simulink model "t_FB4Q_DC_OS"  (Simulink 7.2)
settings: Solver=ode3  SolverMode=SingleTasking  StartTime=0.0  StopTime=0.02  FixedStep=10e-6  MaxStep=5e-6  RelTol=1e-6  AbsTol=1e-6

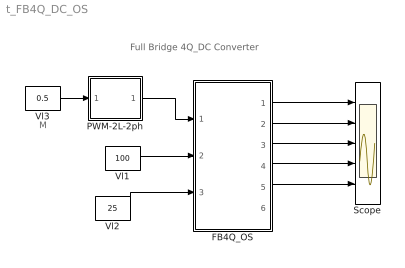
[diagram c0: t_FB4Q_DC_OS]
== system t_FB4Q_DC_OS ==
  note: Full Bridge 4Q_DC Converter
  note: M
  FB4Q_OS : Subsystem  mask{L=5e-3, IL0=30, C=2e-4, VC0=50, R=10}
      mask prompts: L "Inductance L"; IL0 "Initial Current"; C "Cap"; VC0 "Initial Cap Voltage"; R "Load Resistance"
      mask help: Full Bridge 4Q Converter Input Vector u: u[0]= T1.gate u[1]= T2.gate u[2]= T3.gate u[3]= T4.gate u[4]= E.V u[5]= IDC.i Output Vector y: y[0]= T1.I y[1]= D1.I y[2]= T3.I y[3]= D3.I y[4]= Vo.V y[5]= L1.I y[6]= C1.V y[7]= E.I Parameter Vector p: p[0]= L1.L p[1]= L1.iL0 p[2]= C1.C p[3]= C1.vC0 p[4]= R1.r You can pause the simulation during running, change the Parameters you want and continue the Simulation
  PWM-2L-2ph : Subsystem  mask(PWM-2L-2PH){FT=500, PHT=0, DT=1e-6}
      mask prompts: FT "Triangular Frequency"; PHT "Trian. Phase Angle (Degree)"; DT "Dead Time"
  Scope : Scope  NumInputPorts=5
  Vl1 : Constant  Value=100
  Vl2 : Constant  Value=25
  Vl3 : Constant  Value=0.5
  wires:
  FB4Q_OS/1("iT1, iD1") -> Scope/1
  PWM-2L-2ph/1(O1) -> FB4Q_OS/1(sw)
  Vl1/1 -> FB4Q_OS/2(E)
  Vl2/1 -> FB4Q_OS/3(ID)
  FB4Q_OS/4(iL) -> Scope/4
  FB4Q_OS/3(vO) -> Scope/3
  Vl3/1 -> PWM-2L-2ph/1(I1)
  FB4Q_OS/2("iT3, iD3") -> Scope/2
  FB4Q_OS/5(vC) -> Scope/5

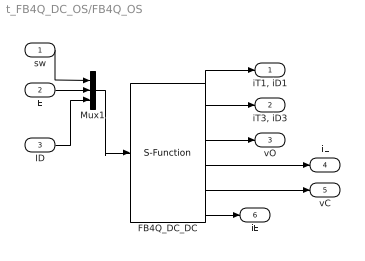
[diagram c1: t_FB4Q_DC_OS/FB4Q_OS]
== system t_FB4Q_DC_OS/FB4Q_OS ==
  sw : Inport  OutDataType=sfix(16)  OutScaling=2^0
  E : Inport  Port=2  OutDataType=sfix(16)  OutScaling=2^0
  ID : Inport  Port=3  OutDataType=sfix(16)  OutScaling=2^0
  FB4Q_DC_DC : S-Function  FunctionName=s_FB4Q_DC_OS  Parameters="[L  IL0  C  VC0   R]"  EnableBusSupport=off
  Mux1 : Mux  Inputs=3
  "iT1, iD1" : Outport  OutDataType=sfix(16)  OutScaling=2^0
  "iT3, iD3" : Outport  Port=2  OutDataType=sfix(16)  OutScaling=2^0
  vO : Outport  Port=3  OutDataType=sfix(16)  OutScaling=2^0
  iL : Outport  Port=4  OutDataType=sfix(16)  OutScaling=2^0
  vC : Outport  Port=5  OutDataType=sfix(16)  OutScaling=2^0
  iE : Outport  Port=6  OutDataType=sfix(16)  OutScaling=2^0
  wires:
  Mux1/1 -> FB4Q_DC_DC/1
  sw/1 -> Mux1/1
  E/1 -> Mux1/2
  FB4Q_DC_DC/1 -> "iT1, iD1"/1
  FB4Q_DC_DC/2 -> "iT3, iD3"/1
  ID/1 -> Mux1/3
  FB4Q_DC_DC/4 -> iL/1
  FB4Q_DC_DC/3 -> vO/1
  FB4Q_DC_DC/5 -> vC/1
  FB4Q_DC_DC/6 -> iE/1

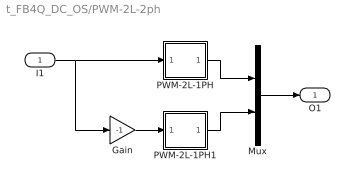
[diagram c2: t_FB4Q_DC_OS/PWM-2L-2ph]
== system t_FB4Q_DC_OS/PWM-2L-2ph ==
  I1 : Inport  OutDataType=sfix(16)  OutScaling=2^0
  Gain : Gain  Gain=-1  ParameterDataType=sfix(16)  ParameterScaling=2^0  OutDataType=sfix(16)  OutScaling=2^0
  Mux : Mux  Inputs=2
  PWM-2L-1PH : Subsystem  mask(PWM-2L-1PH){FT=FT, PHT=PHT, DT=DT}
      mask prompts: FT "Triangular Frequency"; PHT "Trian. Phase Angle (Degree)"; DT "Dead Time"
      mask help: Pulse Width Modulation for 1 Phase Converter
  PWM-2L-1PH1 : Subsystem  mask(PWM-2L-1PH){FT=FT, PHT=PHT, DT=DT}
      mask prompts: FT "Triangular Frequency"; PHT "Trian. Phase Angle (Degree)"; DT "Dead Time"
      mask help: Pulse Width Modulation for 1 Phase Converter
  O1 : Outport
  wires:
  Gain/1 -> PWM-2L-1PH1/1(In1)
  I1/1 -> Gain/1, PWM-2L-1PH/1(In1)
  PWM-2L-1PH/1(Out1) -> Mux/1
  PWM-2L-1PH1/1(Out1) -> Mux/2
  Mux/1 -> O1/1

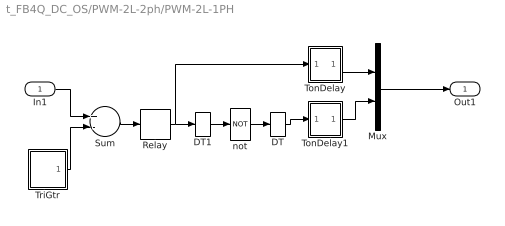
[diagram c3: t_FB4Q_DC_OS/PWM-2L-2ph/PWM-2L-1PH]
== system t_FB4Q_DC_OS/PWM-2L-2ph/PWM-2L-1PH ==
  In1 : Inport  OutDataType=sfix(16)  OutScaling=2^0
  DT : DataTypeConversion
  DT1 : DataTypeConversion
  Mux : Mux  Inputs=2
  Relay : Relay  OutDataType=sfix(16)  OutScaling=2^0
  Sum : Sum  Inputs=+-  OutDataType=sfix(16)  OutScaling=2^0
  TonDelay : Subsystem  mask(TonDelay){DT=DT}
      mask prompts: DT "Dead Time"
      mask help: Turn on dead time to protect against short circuit of the converter leg
  TonDelay1 : Subsystem  mask(TonDelay){DT=DT}
      mask prompts: DT "Dead Time"
      mask help: Turn on dead time to protect against short circuit of the converter leg
  TriGtr : Subsystem  mask(TriGtr){T=1/FT, Td=PHT/FT/360}
      mask prompts: T "Period Time"; Td "Time Delay"
      mask help: Triangular Wave Generator with variable time delay
  not : Logic  Operator=NOT  Inputs=1
  Out1 : Outport  InitialOutput=0
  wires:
  DT1/1 -> not/1
  DT/1 -> TonDelay1/1(s1)
  In1/1 -> Sum/1
  TriGtr/1(O) -> Sum/2
  Sum/1 -> Relay/1
  not/1 -> DT/1
  TonDelay1/1(s1d) -> Mux/2
  Relay/1 -> DT1/1, TonDelay/1(s1)
  TonDelay/1(s1d) -> Mux/1
  Mux/1 -> Out1/1

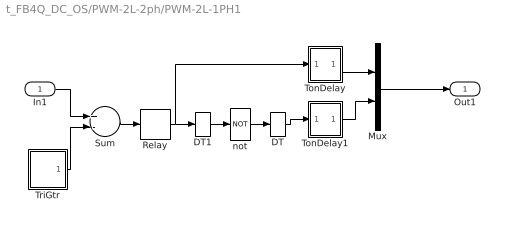
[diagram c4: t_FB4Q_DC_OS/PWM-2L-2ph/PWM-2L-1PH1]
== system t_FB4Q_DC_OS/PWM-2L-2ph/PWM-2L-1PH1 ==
  In1 : Inport  OutDataType=sfix(16)  OutScaling=2^0
  DT : DataTypeConversion
  DT1 : DataTypeConversion
  Mux : Mux  Inputs=2
  Relay : Relay  OutDataType=sfix(16)  OutScaling=2^0
  Sum : Sum  Inputs=+-  OutDataType=sfix(16)  OutScaling=2^0
  TonDelay : Subsystem  mask(TonDelay){DT=DT}
      mask prompts: DT "Dead Time"
      mask help: Turn on dead time to protect against short circuit of the converter leg
  TonDelay1 : Subsystem  mask(TonDelay){DT=DT}
      mask prompts: DT "Dead Time"
      mask help: Turn on dead time to protect against short circuit of the converter leg
  TriGtr : Subsystem  mask(TriGtr){T=1/FT, Td=PHT/FT/360}
      mask prompts: T "Period Time"; Td "Time Delay"
      mask help: Triangular Wave Generator with variable time delay
  not : Logic  Operator=NOT  Inputs=1
  Out1 : Outport  InitialOutput=0
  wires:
  Mux/1 -> Out1/1
  TonDelay/1(s1d) -> Mux/1
  Relay/1 -> TonDelay/1(s1), DT1/1
  TonDelay1/1(s1d) -> Mux/2
  not/1 -> DT/1
  Sum/1 -> Relay/1
  TriGtr/1(O) -> Sum/2
  In1/1 -> Sum/1
  DT/1 -> TonDelay1/1(s1)
  DT1/1 -> not/1

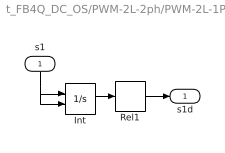
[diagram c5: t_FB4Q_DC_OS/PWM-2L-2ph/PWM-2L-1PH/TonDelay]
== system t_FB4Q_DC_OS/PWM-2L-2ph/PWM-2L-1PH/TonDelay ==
  s1 : Inport  Orientation=down  OutDataType=sfix(16)  OutScaling=2^0
  Int : Integrator  ExternalReset=falling
  Rel1 : Relay  OnSwitchValue=DT  OutDataType=sfix(16)  OutScaling=2^0
  s1d : Outport  InitialOutput=0
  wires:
  Int/1 -> Rel1/1
  s1/1 -> Int/2, Int/1
  Rel1/1 -> s1d/1

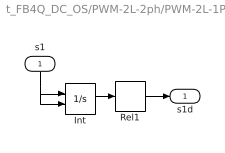
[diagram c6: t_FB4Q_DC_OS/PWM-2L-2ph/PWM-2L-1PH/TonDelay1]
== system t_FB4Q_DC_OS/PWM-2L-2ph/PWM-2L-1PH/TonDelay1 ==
  s1 : Inport  Orientation=down  OutDataType=sfix(16)  OutScaling=2^0
  Int : Integrator  ExternalReset=falling
  Rel1 : Relay  OnSwitchValue=DT  OutDataType=sfix(16)  OutScaling=2^0
  s1d : Outport  InitialOutput=0
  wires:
  Int/1 -> Rel1/1
  s1/1 -> Int/2, Int/1
  Rel1/1 -> s1d/1

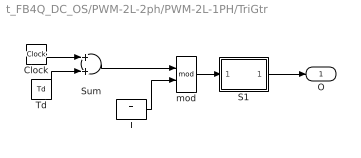
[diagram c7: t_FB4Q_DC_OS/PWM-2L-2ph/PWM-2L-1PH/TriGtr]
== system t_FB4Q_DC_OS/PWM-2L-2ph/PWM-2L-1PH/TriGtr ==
  Clock : Clock
  S1 : Subsystem
  Sum : Sum  OutDataType=sfix(16)  OutScaling=2^0
  T : Constant  Value=T  OutDataType=sfix(16)  OutScaling=2^0
  Td : Constant  Value=Td  OutDataType=sfix(16)  OutScaling=2^0
  mod : Math  Operator=mod
  O : Outport  InitialOutput=0
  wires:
  mod/1 -> S1/1(I1)
  S1/1(O1) -> O/1
  Clock/1 -> Sum/1
  T/1 -> mod/2
  Sum/1 -> mod/1
  Td/1 -> Sum/2

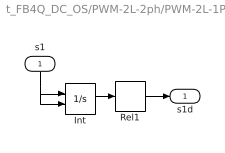
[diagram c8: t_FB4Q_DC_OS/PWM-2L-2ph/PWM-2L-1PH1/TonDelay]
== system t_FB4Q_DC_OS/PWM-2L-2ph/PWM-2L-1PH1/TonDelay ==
  s1 : Inport  Orientation=down  OutDataType=sfix(16)  OutScaling=2^0
  Int : Integrator  ExternalReset=falling
  Rel1 : Relay  OnSwitchValue=DT  OutDataType=sfix(16)  OutScaling=2^0
  s1d : Outport  InitialOutput=0
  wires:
  Rel1/1 -> s1d/1
  s1/1 -> Int/1, Int/2
  Int/1 -> Rel1/1

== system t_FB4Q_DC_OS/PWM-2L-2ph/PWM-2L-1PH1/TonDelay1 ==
  s1 : Inport  Orientation=down  OutDataType=sfix(16)  OutScaling=2^0
  Int : Integrator  ExternalReset=falling
  Rel1 : Relay  OnSwitchValue=DT  OutDataType=sfix(16)  OutScaling=2^0
  s1d : Outport  InitialOutput=0
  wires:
  Rel1/1 -> s1d/1
  s1/1 -> Int/1, Int/2
  Int/1 -> Rel1/1

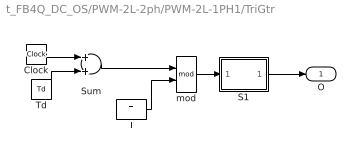
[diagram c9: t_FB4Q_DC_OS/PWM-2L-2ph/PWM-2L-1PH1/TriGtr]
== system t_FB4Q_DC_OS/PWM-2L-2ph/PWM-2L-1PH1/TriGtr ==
  Clock : Clock
  S1 : Subsystem
  Sum : Sum  OutDataType=sfix(16)  OutScaling=2^0
  T : Constant  Value=T  OutDataType=sfix(16)  OutScaling=2^0
  Td : Constant  Value=Td  OutDataType=sfix(16)  OutScaling=2^0
  mod : Math  Operator=mod
  O : Outport  InitialOutput=0
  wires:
  Td/1 -> Sum/2
  Sum/1 -> mod/1
  T/1 -> mod/2
  Clock/1 -> Sum/1
  S1/1(O1) -> O/1
  mod/1 -> S1/1(I1)

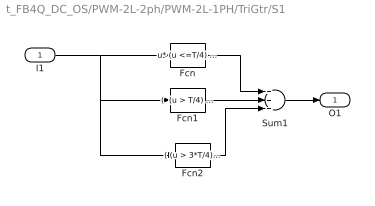
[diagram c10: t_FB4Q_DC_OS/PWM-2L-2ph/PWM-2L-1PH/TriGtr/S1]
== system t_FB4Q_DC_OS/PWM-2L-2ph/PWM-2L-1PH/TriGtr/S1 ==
  I1 : Inport  OutDataType=sfix(16)  OutScaling=2^0
  Fcn : Fcn  Expr=u* (u <=T/4) * 4/T
  Fcn1 : Fcn  Expr="(  (u > T/4) && ( u <=3*T/4) )* ( 1 - (u-T/4) *4/T )"
  Fcn2 : Fcn  Expr=( (u > 3*T/4)&& (u<=T)) * ( ((u -3*T/4)* 4/T )-1 )
  Sum1 : Sum  Inputs=+++  OutDataType=sfix(16)  OutScaling=2^0
  O1 : Outport
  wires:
  Fcn2/1 -> Sum1/3
  Fcn1/1 -> Sum1/2
  Fcn/1 -> Sum1/1
  Sum1/1 -> O1/1
  I1/1 -> Fcn/1, Fcn2/1, Fcn1/1

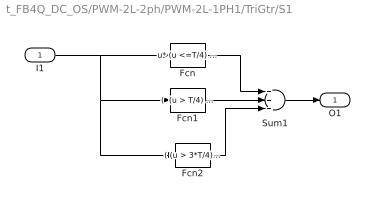
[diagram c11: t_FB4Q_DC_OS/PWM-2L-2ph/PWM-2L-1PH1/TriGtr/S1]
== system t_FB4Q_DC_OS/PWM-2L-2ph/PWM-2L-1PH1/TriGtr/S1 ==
  I1 : Inport  OutDataType=sfix(16)  OutScaling=2^0
  Fcn : Fcn  Expr=u* (u <=T/4) * 4/T
  Fcn1 : Fcn  Expr="(  (u > T/4) && ( u <=3*T/4) )* ( 1 - (u-T/4) *4/T )"
  Fcn2 : Fcn  Expr=( (u > 3*T/4)&& (u<=T)) * ( ((u -3*T/4)* 4/T )-1 )
  Sum1 : Sum  Inputs=+++  OutDataType=sfix(16)  OutScaling=2^0
  O1 : Outport
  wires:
  I1/1 -> Fcn1/1, Fcn2/1, Fcn/1
  Sum1/1 -> O1/1
  Fcn/1 -> Sum1/1
  Fcn1/1 -> Sum1/2
  Fcn2/1 -> Sum1/3
